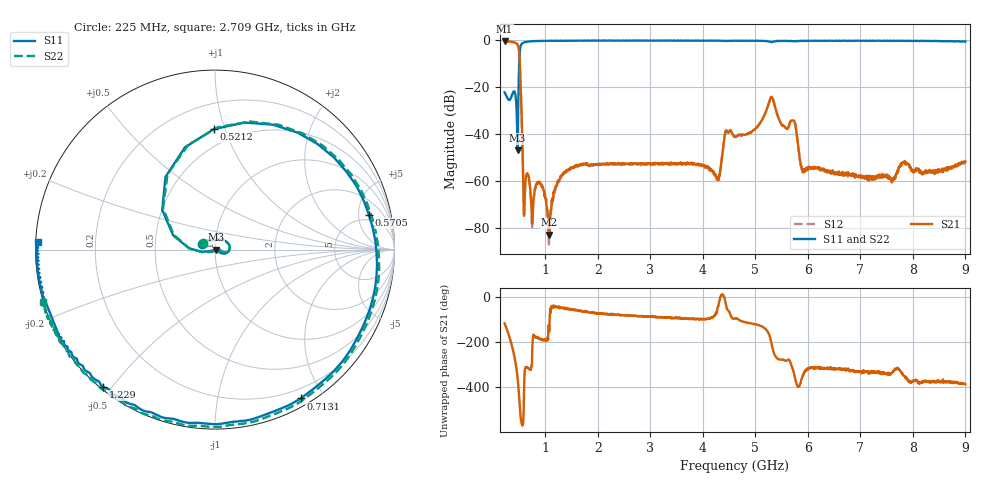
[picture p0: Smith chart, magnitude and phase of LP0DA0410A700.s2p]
!Agilent Technologies,E8358A,US41080443,A.07.50.56
!Agilent E8358A: A.07.50.56
!Date: Wednesday, August 31, 2016 09:04:56
!Correction: S11(Full 2 Port(1,2))
!S21(Full 2 Port(1,2))
!S12(Full 2 Port(1,2))
!S22(Full 2 Port(1,2))
!S2P File: Measurements: S11, S21, S12, S22:
# Hz S  dB  R 50
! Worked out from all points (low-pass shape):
!   1601 points, 225 MHz to 9 GHz, reference 50 ohm
!   highest |S21| = -0.23 dB at 225 MHz (marker M1); lowest = -82.7 dB at 1.075 GHz (marker M2)
!   |S21| within 3 dB of the highest: start of sweep to 493.2 MHz
!   lowest |S11| = -46.7 dB at 471.8 MHz (marker M3), VSWR 1.01, Z = 50.5 - j0.0289 ohm
!   |S11| at or under -10 dB: start of sweep to 502.6 MHz
!   |S22| runs from -41.4 to 0.1 dB; largest |S21 - S12| = 0.021
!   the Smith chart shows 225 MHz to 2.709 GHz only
!   S11 on the Smith chart (normalised r, x): 225 MHz: 0.87, +0.06; 521.2 MHz: 0.38, +0.92; 570.5 MHz: 3.95, +6.75; 713.1 MHz: 0.09, -1.73; 1.229 GHz: 0.01, -0.48; 2.709 GHz: 0.01, +0.02
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2.25e8  -22.10 155.1  -0.23 -117.3  -0.42 -117.0  -21.96 150.7
3.237188e8  -25.27 88.9  -0.43 177.3  -0.62 177.6  -25.11 78.3
3.950156e8  -21.80 21.9  -0.74 114.2  -0.93 114.5  -21.67 21.1
4.717969e8  -46.71 -3.6  -1.81 3.0  -1.99 3.3  -34.44 1.9
5.211562e8  -3.46 90.5  -13.38 -149.7  -13.55 -149.4  -3.32 88.5
5.705156e8  -1.11 12.6  -50.17 153.2  -50.22 153.9  -0.97 11.2
6.143906e8  -0.70 -19.8  -62.84 41.3  -63.40 42.5  -0.57 -20.7
7.131094e8  -0.38 -60.1  -63.54 38.9  -63.15 39.1  -0.25 -60.3
9.050625e8  -0.21 -98.5  -61.04 174.3  -60.59 174.2  -0.07 -98.6
1.075078e9  -0.21 -117.6  -82.72 -152.9  -76.22 -117.6  -0.07 -117.3
1.228641e9  -0.13 -129.2  -61.02 -46.8  -60.96 -45.1  0.01 -129.2
1.689328e9  -0.06 -149.6  -52.64 -63.0  -53.03 -61.3  0.03 -152.1
2.709422e9  -0.11 177.6  -52.51 -83.5  -52.69 -84.0  0.01 -163.1
3.153656e9  -0.12 171.9  -52.54 -89.7  -52.81 -90.7  -0.01 -168.1
4.277953e9  -0.16 159.7  -59.04 -53.9  -58.89 -60.0  -0.01 177.7
4.442484e9  -0.19 156.9  -38.35 -37.5  -38.48 -36.8  -0.09 174.5
4.6125e9  -0.16 155.7  -41.08 -95.4  -41.52 -95.4  -0.03 172.5
5.3145e9  -0.75 144.4  -24.08 146.0  -24.24 146.2  -0.69 158.3
5.901328e9  -0.26 135.1  -54.94 12.1  -56.13 10.7  -0.14 144.7
6.076828e9  -0.14 132.1  -54.31 48.2  -54.09 47.3  -0.08 139.8
7.541156e9  -0.22 116.2  -57.60 19.0  -58.67 26.0  -0.12 110.5
9e9  -0.45 91.9  -51.60 -26.5  -51.63 -24.0  -0.24 83.7
